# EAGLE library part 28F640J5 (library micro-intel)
MICROCOMPUTER/PERIPHERAL DEVICE
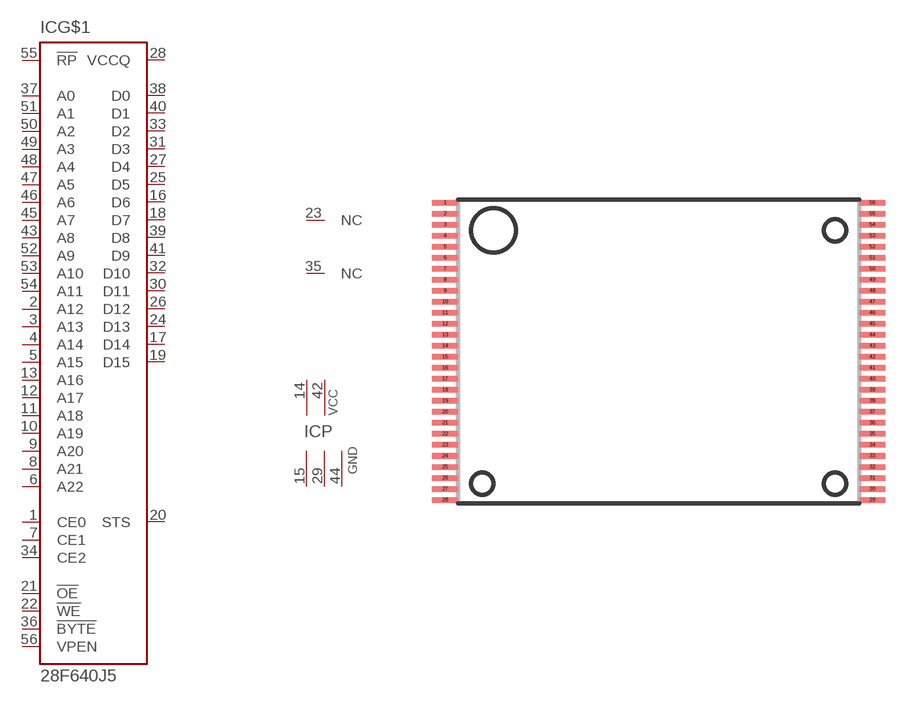
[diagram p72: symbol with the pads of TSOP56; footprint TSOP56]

Designator prefix IC; gates G$1=28F640J5 NC1=NC NC2=NC P=2VCC3GND

## 28F640J5 (OC_FARNELL: unknown; OC_NEWARK: unknown)  [TSOP56]
1  G$1:CE0  in
2  G$1:A12  in
3  G$1:A13  in
4  G$1:A14  in
5  G$1:A15  in
6  G$1:A22  in
7  G$1:CE1  in
8  G$1:A21  in
9  G$1:A20  in
10  G$1:A19  in
11  G$1:A18  in
12  G$1:A17  in
13  G$1:A16  in
14  P:VCC  pwr
15  P:GND  pwr
16  G$1:D6  hiz
17  G$1:D14  hiz
18  G$1:D7  hiz
19  G$1:D15  hiz
20  G$1:STS  out
21  G$1:!OE  in
22  G$1:!WE  in
23  NC1:NC  nc
24  G$1:D13  hiz
25  G$1:D5  hiz
26  G$1:D12  hiz
27  G$1:D4  hiz
28  G$1:VCCQ  pwr
29  P:GND  pwr
30  G$1:D11  hiz
31  G$1:D3  hiz
32  G$1:D10  hiz
33  G$1:D2  hiz
34  G$1:CE2  in
35  NC2:NC  nc
36  G$1:!BYTE  out
37  G$1:A0  in
38  G$1:D0  hiz
39  G$1:D8  hiz
40  G$1:D1  hiz
41  G$1:D9  hiz
42  P:VCC  pwr
43  G$1:A8  in
44  P:GND  pwr
45  G$1:A7  in
46  G$1:A6  in
47  G$1:A5  in
48  G$1:A4  in
49  G$1:A3  in
50  G$1:A2  in
51  G$1:A1  in
52  G$1:A9  in
53  G$1:A10  in
54  G$1:A11  in
55  G$1:!RP  in
56  G$1:VPEN  out

## Footprint TSOP56 (pad centres in mm)
Thin Small Outline Package
smd 1.2 x 0.25: 1 -9.7,6.75; 2 -9.7,6.25; 3 -9.7,5.75; 4 -9.7,5.25; 5 -9.7,4.75; 6 -9.7,4.25; 7 -9.7,3.75; 8 -9.7,3.25; 9 -9.7,2.75; 10 -9.7,2.25; 11 -9.7,1.75; 12 -9.7,1.25; 13 -9.7,0.75; 14 -9.7,0.25; 15 -9.7,-0.25; 16 -9.7,-0.75; 17 -9.7,-1.25; 18 -9.7,-1.75; 19 -9.7,-2.25; 20 -9.7,-2.75; 21 -9.7,-3.25; 22 -9.7,-3.75; 23 -9.7,-4.25; 24 -9.7,-4.75; 25 -9.7,-5.25; 26 -9.7,-5.75; 27 -9.7,-6.25; 28 -9.7,-6.75; 29 9.7,-6.75; 30 9.7,-6.25; 31 9.7,-5.75; 32 9.7,-5.25; 33 9.7,-4.75; 34 9.7,-4.25; 35 9.7,-3.75; 36 9.7,-3.25; 37 9.7,-2.75; 38 9.7,-2.25; 39 9.7,-1.75; 40 9.7,-1.25; 41 9.7,-0.75; 42 9.7,-0.25; 43 9.7,0.25; 44 9.7,0.75; 45 9.7,1.25; 46 9.7,1.75; 47 9.7,2.25; 48 9.7,2.75; 49 9.7,3.25; 50 9.7,3.75; 51 9.7,4.25; 52 9.7,4.75; 53 9.7,5.25; 54 9.7,5.75; 55 9.7,6.25; 56 9.7,6.75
